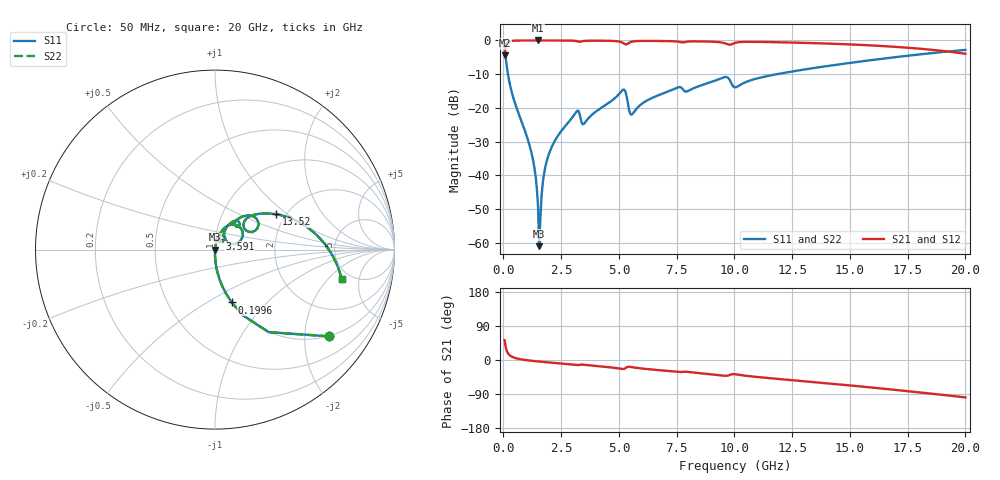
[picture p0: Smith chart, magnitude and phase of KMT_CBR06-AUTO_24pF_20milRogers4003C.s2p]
! Data measured by Modelithics Inc. support@modelithics.com 813-866-6335
! KEMET CBR06-AUTO 24pF, Pad Width= 0.851mm, Pad Length= 0.64mm, Pad Gap= 0.62mm, 20mil Rogers 4003C substrate Data, January 2022
# hz S ma R 50
! 2 Port Network Data from SP1.SP block
! freq  magS11  angS11  magS21  angS21  magS12  angS12  magS22  angS22
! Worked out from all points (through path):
!   401 points, 50 MHz to 20 GHz, reference 50 ohm
!   highest |S21| = -0.01 dB at 1.496 GHz (marker M1); lowest = -4.4 dB at 50 MHz (marker M2)
!   group delay of S21, straight-line fit = 14 ps
!   lowest |S11| = -61.0 dB at 1.546 GHz (marker M3), VSWR 1.00, Z = 50.1 - j0.0687 ohm
!   |S11| at or under -10 dB: 194.8 MHz to 11.84 GHz (11.64 GHz wide, 194 % of centre)
!   |S22| runs from -61.0 to -2.0 dB; largest |S21 - S12| = 0
!   S11 on the Smith chart (normalised r, x): 50 MHz: 0.99, -2.62; 199.6 MHz: 0.99, -0.65; 3.591 GHz: 1.04, +0.13; 13.52 GHz: 1.78, +0.83; 20 GHz: 4.19, -2.88
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5e7  0.7959 -37.4  0.6051 52.6  0.6051 52.6  0.7959 -37.4
1.99625e8  0.3085 -72.5  0.9509 17.4  0.9509 17.4  0.3085 -72.5
4.98875e8  0.1178 -84.4  0.9926 5.4  0.9926 5.4  0.1178 -84.4
1.197125e9  0.0228 -90.5  0.9992 -1.9  0.9992 -1.9  0.0228 -90.5
1.34675e9  0.01257 -90.2  0.9993 -2.9  0.9993 -2.9  0.01257 -90.2
1.496375e9  0.003527 -83.8  0.9993 -3.8  0.9993 -3.8  0.003527 -83.8
1.54625e9  0.0008955 -50.0  0.9993 -4.1  0.9993 -4.1  0.0008955 -50.0
1.646e9  0.004827 77.6  0.9993 -4.7  0.9993 -4.7  0.004827 77.6
1.795625e9  0.01247 81.3  0.9992 -5.5  0.9992 -5.5  0.01247 81.3
2.094875e9  0.02671 81.2  0.9988 -7.1  0.9988 -7.1  0.02671 81.2
3.14225e9  0.08655 66.1  0.9803 -13.2  0.9803 -13.2  0.08655 66.1
3.391625e9  0.05974 48.2  0.9688 -12.0  0.9688 -12.0  0.05974 48.2
3.591125e9  0.0648 68.2  0.9882 -13.2  0.9882 -13.2  0.0648 68.2
5.13725e9  0.1811 49.7  0.9326 -23.6  0.9326 -23.6  0.1811 49.7
5.586125e9  0.08111 46.7  0.9637 -19.1  0.9637 -19.1  0.08111 46.7
6.73325e9  0.1555 61.2  0.9821 -26.8  0.9821 -26.8  0.1555 61.2
9.576125e9  0.2865 38.4  0.9098 -41.7  0.9098 -41.7  0.2865 38.4
1.0025e10  0.2018 34.5  0.9189 -37.5  0.9189 -37.5  0.2018 34.5
1.336662e10  0.3866 30.9  0.9135 -57.9  0.9135 -57.9  0.3866 30.9
1.351625e10  0.3936 30.0  0.9104 -58.7  0.9104 -58.7  0.3936 30.0
1.670825e10  0.5515 10.7  0.8146 -77.3  0.8146 -77.3  0.5515 10.7
2e10  0.7241 -13.1  0.6345 -98.6  0.6345 -98.6  0.7241 -13.1
